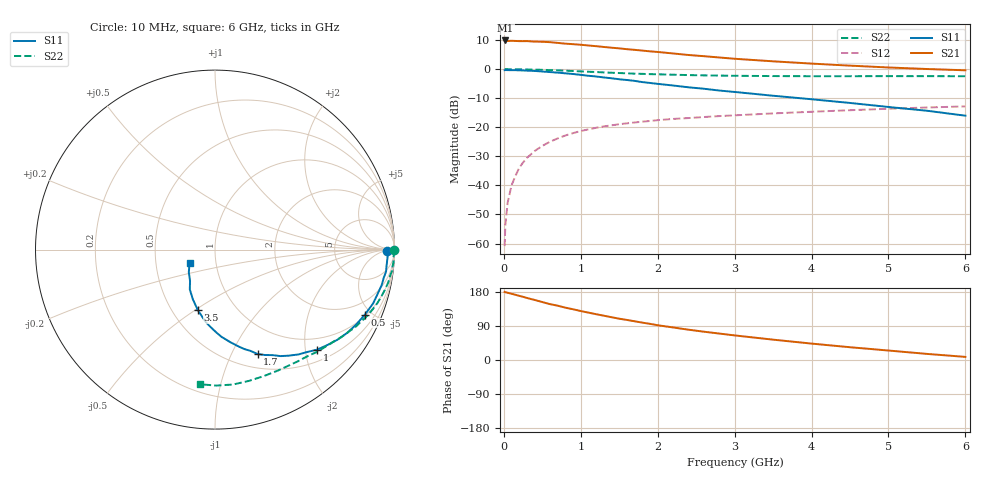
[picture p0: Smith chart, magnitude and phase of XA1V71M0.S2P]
! SIEMENS Discrete & RF Semiconductors
! BFY180
! Si NPN RF Bipolar Junction Transistor in MICRO-X
! VCE = 1.75 V  IC = 1 mA
! Common Emitter S-Parameters:  May  1997
# GHz  S  MA  R  50
!  f  S11  S21  S12  S22
! GHz  MAG  ANG  MAG  ANG  MAG  ANG  MAG  ANG
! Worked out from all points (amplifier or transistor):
!   36 points, 10 MHz to 6 GHz, reference 50 ohm
!   highest |S21| = 9.9 dB at 20 MHz (marker M1)
!   |S21| within 3 dB of that: start of sweep to 1.598 GHz
!   unconditionally stable (mu >= 1): 3.534 GHz to end of sweep
!   at 250 MHz: K = 0.09, MSG = 20.9 dB, |S12| = -32.1 dB
!   at 1.4 GHz: K = 0.54, MSG = 13.4 dB, |S12| = -19.3 dB
!   at 6 GHz: K = 1.08, MAG = 4.5 dB, |S12| = -12.8 dB
!   S11 on the Smith chart (normalised r, x): 10 MHz: 49, -9; 500 MHz: 1.08, -4.58; 1 GHz: 0.74, -2.25; 1.7 GHz: 0.66, -1.26; 3.5 GHz: 0.67, -0.51; 6 GHz: 0.75, -0.11
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0.01  0.9609 -0.4  3.065 179.7  0.0009 90.2  0.9974 -0.2
0.02  0.9646 -0.9  3.115 178.8  0.0021 92.1  0.9999 -0.6
0.05  0.9626 -2.3  3.047 177.5  0.0051 86.5  0.9982 -1.4
0.1  0.9603 -4.9  3.074 174.8  0.01 86.0  0.994 -2.7
0.15  0.9607 -7.4  3.055 172.1  0.0145 85.4  0.9972 -4.1
0.2  0.9531 -9.5  3.032 169.3  0.02 84.7  0.9932 -5.5
0.3  0.9424 -14.1  3.036 163.7  0.0297 80.1  0.9874 -8.2
0.5  0.9107 -23.4  2.959 152.9  0.0478 73.5  0.9724 -13.4
0.6  0.891 -27.9  2.911 147.4  0.0564 70.6  0.9624 -15.9
0.8  0.8469 -36.4  2.744 138.1  0.0722 64.8  0.9398 -20.7
1  0.7975 -44.3  2.627 129.2  0.0862 59.6  0.9152 -25.1
1.1  0.7691 -47.8  2.552 125.0  0.092 57.3  0.9025 -27.1
1.4  0.6967 -58.4  2.338 112.9  0.1079 50.8  0.8671 -32.8
1.7  0.6281 -67.8  2.148 102.2  0.1208 46.1  0.836 -37.8
2  0.5579 -76.0  1.975 91.7  0.1325 41.8  0.8149 -42.4
2.2  0.5229 -80.6  1.861 85.9  0.1391 39.0  0.8028 -45.5
2.4  0.4871 -85.8  1.751 80.0  0.144 37.0  0.7895 -48.2
2.8  0.4287 -93.8  1.587 69.8  0.1557 33.3  0.775 -53.4
3.5  0.3486 -106.1  1.363 53.7  0.1731 27.5  0.7597 -62.4
4.5  0.262 -122.4  1.149 33.7  0.1965 19.6  0.7555 -75.5
5.5  0.1924 -139.4  1.005 16.1  0.2188 11.8  0.7576 -89.4
6  0.1582 -152.9  0.955 8.2  0.2287 7.6  0.7551 -96.4
